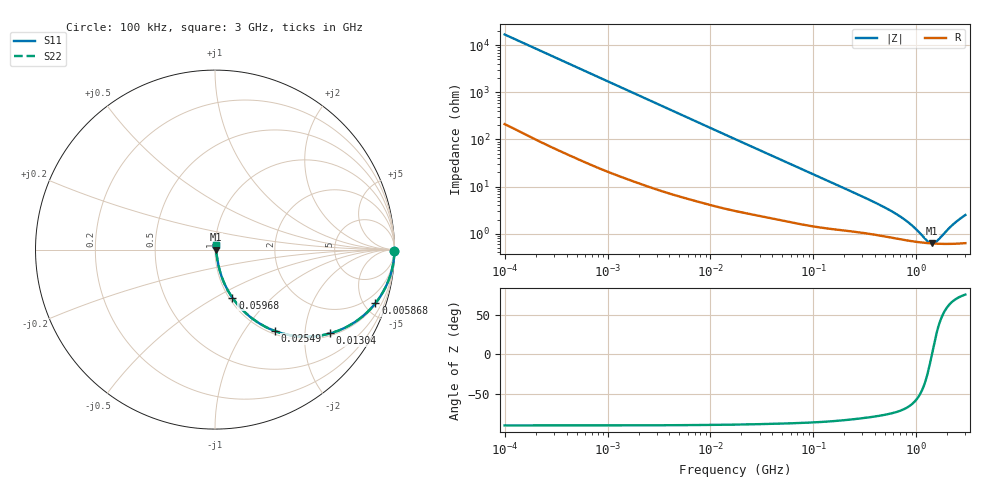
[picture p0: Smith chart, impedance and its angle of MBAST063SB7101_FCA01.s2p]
! MBAST063SB7101_FCA01  S-PARAMETER MODEL  ( Standard Model )
! Model Generated by TAIYO YUDEN Corporation (http://www.ty-top.com)
! Version 2.0
! TAIYO YUDEN Control No. 231201
! Copyright(c) 2020 TAIYO YUDEN CO.,LTD. All Rights Reserved.
! Product Description (link to TY-COMPAS)
! https://ds.yuden.co.jp/TYCOMPAS/or/detail?pn=MBAST063SB7101KFCA01&u=M
! Products Name : Multilayer Ceramic Capacitors
! Characteristics :
!  Capacitance : 100 [pF] , Rated Voltage : 25 [V] , TCC : X7R
!  Case Size : 0.6 x 0.3 / 0.024 x 0.012 [mm/inch] , Thickness : 0.3 / 0.012 [mm/inch]
!  (Conditions: Temperature = 25 [degC] , DC Bias Voltage = 0 [V])
! External Node Assignments :
!  1  o---| |---o  2
! GND o---------o GND
! Frequency Range : 100kHz  -  3GHz  [ 401 STEP ]
# MHZ S RI R 50
! Freq[MHz].  S11 Real  S11 Imag  S21 Real  S21 Imag  S12 Real  S12 Imag  S22 Real  S22 Imag
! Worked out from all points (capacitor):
!   401 points, 100 kHz to 3 GHz, reference 50 ohm
!   read as one part in series: C = 93.7 pF near 105.3 kHz
!   lowest |Z| = 621 mohm at 1.421 GHz (marker M1)
!   series resonance near 1.418 GHz, so ESL is about 130 pH
!   S11 on the Smith chart (normalised r, x): 100 kHz: open; 5.868 MHz: 1.11, -5.95; 13.04 MHz: 1.07, -2.70; 25.49 MHz: 1.05, -1.39; 59.68 MHz: 1.04, -0.60; 3 GHz: 1.01, +0.05
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0.1  0.9999 -0.0059  0.000109 0.0059  0.000109 0.0059  0.9999 -0.0059
0.562235  0.9986 -0.0327  0.00145 0.0327  0.00145 0.0327  0.9986 -0.0327
1.458987  0.9919 -0.0837  0.00815 0.0837  0.00815 0.0837  0.9919 -0.0837
3.161081  0.9654 -0.1753  0.0346 0.1753  0.0346 0.1753  0.9654 -0.1753
5.867632  0.894 -0.2986  0.106 0.2986  0.106 0.2986  0.894 -0.2986
8.636841  0.7993 -0.3898  0.2007 0.3898  0.2007 0.3898  0.7993 -0.3898
13.04487  0.6418 -0.4667  0.3582 0.4667  0.3582 0.4667  0.6418 -0.4667
17.7727  0.4969 -0.4851  0.5031 0.4851  0.5031 0.4851  0.4969 -0.4851
25.49486  0.3322 -0.453  0.6678 0.453  0.6678 0.453  0.3322 -0.453
38.50681  0.1883 -0.3686  0.8117 0.3686  0.8117 0.3686  0.1883 -0.3686
59.67813  0.0967 -0.2679  0.9033 0.2679  0.9033 0.2679  0.0967 -0.2679
97.38194  0.0464 -0.1752  0.9536 0.1752  0.9536 0.1752  0.0464 -0.1752
205.6221  0.019 -0.086  0.981 0.086  0.981 0.086  0.019 -0.086
547.5153  0.00925 -0.0303  0.9908 0.0303  0.9908 0.0303  0.00925 -0.0303
826.9535  0.00735 -0.016  0.9926 0.016  0.9926 0.016  0.00735 -0.016
990.4458  0.0068 -0.0105  0.9932 0.0105  0.9932 0.0105  0.0068 -0.0105
1281.618  0.00629 -0.00292  0.9937 0.00292  0.9937 0.00292  0.00629 -0.00292
1420.79  0.00617 6.36e-05  0.9938 -6.36e-05  0.9938 -6.36e-05  0.00617 6.36e-05
1575.075  0.0061 0.00306  0.9939 -0.00306  0.9939 -0.00306  0.0061 0.00306
2259.438  0.00625 0.0141  0.9937 -0.0141  0.9937 -0.0141  0.00625 0.0141
2706.139  0.00657 0.0201  0.9934 -0.0201  0.9934 -0.0201  0.00657 0.0201
3000  0.00684 0.0239  0.9932 -0.0239  0.9932 -0.0239  0.00684 0.0239
